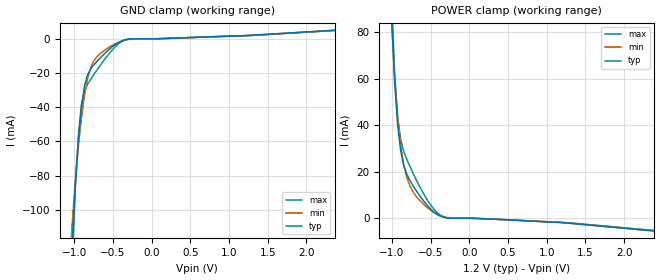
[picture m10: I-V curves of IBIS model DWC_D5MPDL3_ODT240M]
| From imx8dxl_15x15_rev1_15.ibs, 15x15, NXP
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[Model] DWC_D5MPDL3_ODT240M
Model_type   Input
Polarity   Non-Inverting
Enable   Active-High
C_comp   1.454pF   1.360pF   1.566pF
C_comp_power_clamp   328.991fF   303.140fF   352.537fF
C_comp_gnd_clamp 1.092pF   1.014pF   1.189pF
Vinh = 735.000mV
Vinl = 465.000mV
[Model Spec]
D_overshoot_ampl_h 0.35 NA   NA
D_overshoot_ampl_l 0.35 NA   NA
D_overshoot_area_l 100.000p NA   NA
D_overshoot_area_h 100.000p NA   NA
[Receiver Thresholds]
Vcross_low = 480.000mV
Vcross_high = 720.000mV
Vdiff_ac = 270.000mV
Vdiff_dc = 200.000mV
Tdiffslew_ac = 10.000ns
[Temperature Range]   25.000   125.000   -40.000
[Voltage Range]   1.200V   1.140V   1.300V
[GND Clamp Reference]   0.00V   0.00V   0.00V
[C Comp Corner]
| variable   typ   min   max
C_comp 1.454pF   1.566pF   1.360pF
C_comp_pullup 328.991fF   352.537fF   303.140fF
C_comp_pulldown 1.092pF   1.189pF   1.014pF
[POWER Clamp Reference]   1.200V   1.140V   1.300V
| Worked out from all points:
|   GND clamp passes 1 mA (typ) near -0.37 V on its own axis
|   POWER clamp passes 1 mA (typ) near -0.38 V on its own axis
[GND Clamp]
-1.182V   -342.6mA   -255.5mA   -432.7mA
-1.064V   -160.7mA   -136.1mA   -185.6mA
-1.024V   -117.9mA   -106.7mA   -128.8mA
-984.8mV  -84.28mA   -82.29mA   -86.36mA
-945.5mV  -58.47mA   -62.29mA   -56.38mA
-906.1mV  -39.51mA   -45.96mA   -38.29mA
-866.7mV  -27.35mA   -32.97mA   -30.29mA
-787.9mV  -17.63mA   -16.92mA   -23.67mA
-630.3mV  -9.592mA   -7.405mA   -13.36mA
-433.3mV  -2.26mA    -2.067mA   -3.071mA
-315.2mV  -233uA     -429.7uA   -213.1uA
2.364V    5.063mA    5.035mA    4.889mA
[Power Clamp]
-1.164V   310.6mA    240.7mA    379.9mA
-1.006V   87.98mA    84.72mA    95.87mA
-966.7mV  58.68mA    60.73mA    62.28mA
-927.3mV  40.08mA    43.33mA    43.35mA
-887.9mV  28.93mA    31.24mA    33.72mA
-848.5mV  22.58mA    23.02mA    28.72mA
-809.1mV  18.86mA    17.53mA    25.33mA
-690.9mV  12mA       9.527mA    16.78mA
-493.9mV  3.691mA    3.22mA     5.361mA
-375.8mV  891.1uA    1.045mA    1.292mA
-257.6mV  25.54uA    139.7uA    28.87uA
2.382V    -5.51mA    -5.464mA   -5.297mA
